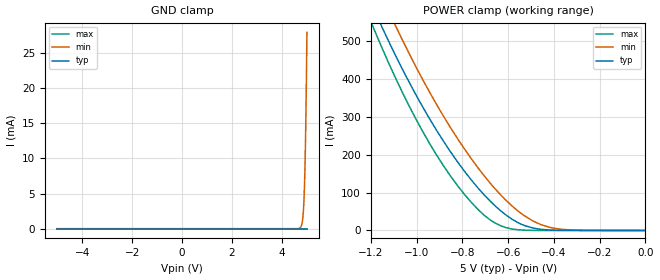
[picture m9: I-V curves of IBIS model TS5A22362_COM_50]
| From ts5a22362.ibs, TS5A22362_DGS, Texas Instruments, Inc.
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[Model]   TS5A22362_COM_50
Model_type  Terminator
| variable   typ   min   max
C_comp   171.53pF   112.61pF   212.00pF
| C_tri-state   171.53pF   112.61pF   212.00pF
[Temperature Range]   40   100   -40
| Ambient temperature   25   85   -40
[Voltage range]   5   4.5   5.5
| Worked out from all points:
|   POWER clamp passes 1 mA (typ) near -0.41 V on its own axis
[GND Clamp]
| TS5A22362_COM_50
|   Voltage   I(typ)   I(min)   I(max)
-5V       -17.05nA   -1.163uA   -6.101nA
4.725V    6.173nA    113uA      4.779nA
4.785V    6.259nA    490.5uA    4.843nA
4.83V     6.324nA    1.37mA     4.892nA
4.865V    6.38nA     2.909mA    4.93nA
4.895V    6.438nA    5.315mA    4.962nA
4.91V     6.476nA    7.052mA    4.978nA
4.925V    6.529nA    9.222mA    4.994nA
4.95V     6.681nA    13.93mA    5.021nA
4.975V    7.025nA    20.14mA    5.048nA
4.985V    7.275nA    23.06mA    5.059nA
5V        7.874nA    27.92mA    5.075nA
[POWER Clamp]
| TS5A22362_COM_50
|   Voltage   I(typ)   I(min)   I(max)
-5V       11.29A     11.24A     12.59A
-1.185V   582.9mA    665.1mA    531mA
-1.155V   542.9mA    624mA      488.2mA
-1.095V   466.6mA    545.2mA    407.1mA
-1.065V   430.3mA    507.5mA    368.9mA
-980mV    334mA      406.7mA    269.2mA
-855mV    210.9mA    275.2mA    146.7mA
-760mV    132.9mA    189mA      73.71mA
-660mV    66.81mA    112.3mA    20.75mA
-530mV    13.33mA    39.33mA    855.5uA
-415mV    1.071mA    7.724mA    15uA
0V        0A         0A         0A
